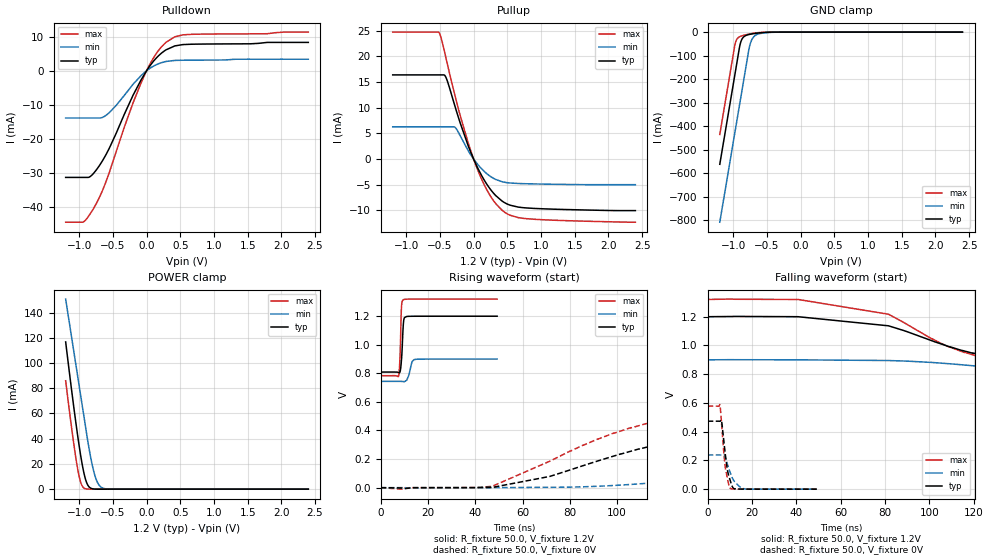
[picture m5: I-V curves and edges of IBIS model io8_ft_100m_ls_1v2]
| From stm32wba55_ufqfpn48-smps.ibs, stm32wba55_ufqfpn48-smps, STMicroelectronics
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[Model]   io8_ft_100m_ls_1v2
Model_type I/O
Polarity   Non-Inverting
Enable   Active-Low
| CAP_THRESHOLD on pad IOFT is "UDTCAPC" :
| Rising=30.0% of vddiom   Falling=70.0% of vddiom
| C_comp min and max val. don't necessarily correlate with the min and max pvt
| but are the smallest and greatest pad capacitance found.
| var   typ   min   max
C_comp   1.75100pF  1.57486pF  1.87844pF
|C_comp_pullup   1.05585pF  962.11500fF  1.08715pF
|C_comp_pulldown   695.15000fF  612.74000fF  791.29000fF
Vinl = 450.0mV
Vinh = 660.0mV
Vmeas = 600.0mV   | Reference voltage for timing measurements
Cref  = 50.0pF   | Timing specification test load capacitance value
Rref  = 1.0MOhm   | Timing specification test load resistance value
Vref  = 660.0mV   | Timing specification test load voltage
[Model Spec]
| TIME_THRESHOLD on pin ZIV11 is "CMOS" :
| Rising=50.0% of vdd   Falling=50.0% of vdd
Vinl 441.50000mV 347.50000mV 471.50000mV
Vinh 755.50000mV 552.50000mV 842.50000mV
| variable   typ   min   max
[Temperature Range] 25.0 140.0 -40.0
| variable   typ   min   max
[Voltage Range] 1.2V 900.0mV 1.32V
| variable   typ   min   max
[POWER Clamp Reference] 1.2V 900.0mV 1.32V
| variable   typ   min   max
[GND Clamp Reference] 0V 0V 0V
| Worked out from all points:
|   slope of the pulldown table from 0 to 0.18 V, typ, clamps not added: 40.6 ohm
|   slope of the pullup table from 0 to 0.18 V, typ, clamps not added: 39.4 ohm
|   GND clamp passes 1 mA (typ) near -0.51 V on its own axis
|   POWER clamp passes 1 mA (typ) near -0.83 V on its own axis
|   rising waveform, R_fixture 50.0, V_fixture 1.2V: 20-80 % time 741ps typ, 1.44ns min, 565ps max; typ from 0.809 V to 1.2 V
|   falling waveform, R_fixture 50.0, V_fixture 1.2V: 20-80 % time 58.6ns typ, 91ns min, 49.9ns max; typ from 1.2 V to 0.809 V
|   rising waveform, R_fixture 50.0, V_fixture 0V: 20-80 % time 69.7ns typ, 118ns min, 54.2ns max; typ from 0 V to 0.473 V
|   falling waveform, R_fixture 50.0, V_fixture 0V: 20-80 % time 2.49ns typ, 3.86ns min, 2.13ns max; typ from 0.473 V to 0 V
[POWER Clamp]
-1.2V     116.7mA    150.7mA    85.92mA
-1.06V    57.23mA    102.6mA    28.68mA
-1.02V    41.75mA    88.91mA    15.5mA
-980mV    27.6mA     75.18mA    5.935mA
-920mV    10.75mA    54.6mA     597.6uA
-870mV    3.065mA    37.68mA    60.82uA
-820mV    594.6uA    22.85mA    5.912uA
-770mV    99.71uA    11.47mA    572nA
-730mV    23.34uA    5.552mA    88.29nA
-680mV    3.779uA    1.833mA    8.565nA
-510mV    7.889nA    23.13uA    53.67pA
2.4V      0A         0A         0A
[GND Clamp]
-1.2V     -561.6mA   -807.5mA   -434.8mA
-980mV    -187.6mA   -433.5mA   -60.76mA
-960mV    -153.6mA   -399.5mA   -38.21mA
-900mV    -54.17mA   -297.5mA   -18.87mA
-870mV    -29.55mA   -246.5mA   -15.73mA
-830mV    -17.05mA   -178.5mA   -12.57mA
-760mV    -9.921mA   -62.77mA   -8.045mA
-730mV    -8.191mA   -35.56mA   -6.403mA
-680mV    -5.826mA   -15.57mA   -4.089mA
-580mV    -2.43mA    -5.043mA   -1.157mA
-330mV    -11.72uA   -245.5uA   -300.5nA
2.4V      872pA      1.056uA    338.3pA
| variable   typ   min   max
[Pullup Reference] 1.2V 900.0mV 1.32V
| variable   typ   min   max
[Pulldown Reference] 0V 0V 0V
[Pullup]
-1.2V     16.39mA    6.276mA    24.72mA
-510mV    16.39mA    6.276mA    24.58mA
-470mV    16.39mA    6.276mA    23.01mA
-410mV    15.89mA    6.276mA    19.68mA
-270mV    10mA       6.109mA    12.02mA
-80mV     2.58mA     1.624mA    3.14mA
10mV      -297.9uA   -180.5uA   -364.9uA
120mV     -3.232mA   -1.915mA   -3.953mA
230mV     -5.55mA    -3.196mA   -6.777mA
450mV     -8.417mA   -4.493mA   -10.26mA
790mV     -9.528mA   -4.811mA   -11.62mA
2.4V      -10.04mA   -4.994mA   -12.3mA
[Pulldown]
-1.2V     -31.2mA    -13.81mA   -44.3mA
-940mV    -31.2mA    -13.81mA   -44.26mA
-850mV    -31.11mA   -13.81mA   -42.26mA
-760mV    -29.39mA   -13.81mA   -39.38mA
-660mV    -26.52mA   -13.68mA   -35.32mA
-550mV    -22.55mA   -12.17mA   -29.6mA
-330mV    -12.74mA   -7.204mA   -16.5mA
-80mV     -2.622mA   -1.37mA    -3.49mA
100mV     2.727mA    1.319mA    3.679mA
290mV     6.144mA    2.737mA    8.347mA
540mV     7.674mA    3.096mA    10.53mA
2.4V      8.312mA    3.389mA    11.33mA
[Ramp]
dV/dt_r 283.797mV/67.15411ns 142.76779mV/117.19779ns 346.62035mV/52.54985ns
dV/dt_f 234.65953mV/57.93901ns 93.75812mV/89.43894ns 321.77274mV/49.4972ns
R_load = 50.0
| Removed startup time: 0s 0s 0s  .
| Removed end time: 49.25ns.
[Rising Waveform]
R_fixture   = 50.0
V_fixture   = 1.2V
V_fixture_min = 900.0mV
V_fixture_max = 1.32V
0s        808.9mV    743.7mV    783.7mV
7.6ns     805.8mV    743.8mV    781mV
7.9ns     804.2mV    743.8mV    820.8mV
8.25ns    813.1mV    743.7mV    931.6mV
8.65ns    860.7mV    743.6mV    1.184V
8.85ns    900.7mV    743.5mV    1.268V
9.6ns     1.14V      742.6mV    1.315V
10.1ns    1.19V      741.9mV    1.318V
14.1ns    1.2V       895.9mV    1.32V
49.25ns   1.2V       899.9mV    1.32V
| Removed startup time: 0s 0s 0s  .
| Removed end time: 1.9992us.
[Falling Waveform]
R_fixture   = 50.0
V_fixture   = 1.2V
V_fixture_min = 900.0mV
V_fixture_max = 1.32V
0s        1.2V       900mV      1.32V
40.8ns    1.2V       900mV      1.32V
81.6ns    1.137V     895.1mV    1.217V
105.7ns   1.009V     876.6mV    1.011V
115.8ns   961.1mV    863.8mV    950.7mV
128.8ns   919.6mV    845.3mV    899.2mV
160.5ns   860.9mV    804.4mV    833.4mV
204ns     828.6mV    774.5mV    800.3mV
408ns     809.1mV    745.2mV    783.8mV
1.999us   808.9mV    743.7mV    783.7mV
| Removed startup time: 0s 0s 0s  .
| Removed end time: 1.99925us.
[Rising Waveform]
R_fixture   = 50.0
V_fixture   = 0V
V_fixture_min = 0V
V_fixture_max = 0V
0s        4.648nV    985.6nV    3.924nV
47.2ns    1.581mV    159.8uV    9.534mV
71.55ns   78.66mV    2.175mV    185.3mV
91.85ns   187.2mV    9.572mV    340.9mV
126.2ns   335.2mV    49.63mV    495.2mV
163.2ns   417.8mV    106.1mV    553.7mV
205.6ns   454.7mV    159.6mV    572.2mV
285.6ns   470.5mV    212.4mV    577.4mV
462.7ns   473.1mV    236.8mV    577.7mV
1.999us   473mV      237.9mV    577.7mV
| Removed startup time: 0s 0s 0s  .
| Removed end time: 49.25ns.
[Falling Waveform]
R_fixture   = 50.0
V_fixture   = 0V
V_fixture_min = 0V
V_fixture_max = 0V
0s        473mV      238mV      577.7mV
5.55ns    472.5mV    238mV      586.8mV
6.3ns     471.2mV    237.8mV    453.6mV
7.2ns     349.2mV    242.8mV    272.6mV
7.9ns     251mV      224.2mV    159.2mV
9.05ns    122.5mV    167mV      64.4mV
10.2ns    59.08mV    114mV      6.034mV
11.65ns   6.073mV    62.72mV    1.607mV
16.1ns    383.8uV    3.927mV    210.4uV
49.25ns   96.56uV    51.16uV    99.89uV
